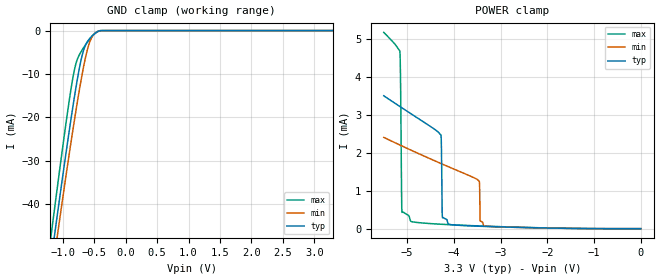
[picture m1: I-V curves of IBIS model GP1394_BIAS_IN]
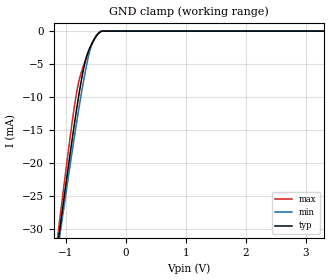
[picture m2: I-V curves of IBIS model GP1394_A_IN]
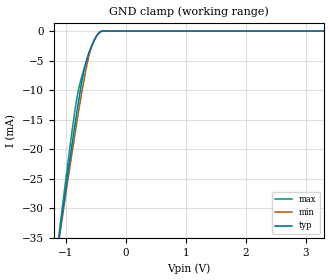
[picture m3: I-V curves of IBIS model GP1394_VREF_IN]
| TEXAS INSTRUMENTS INCORPORATED
| Standard Linear and Logic Group
| IBIS Model of SN74GTLP1394
| 2-Bit LVTTL-TO-GTLP Adjustable-Edge-Rate Bus Tran. with Split LVTTL Port
| This file contains package information for the following:
|  SOIC 16-pin (D) package as [Component] GTLP1394_D
|  TSSOP 16 pin (PW)  package as [Component] GTLP1394_PW
|  TVSOP 16 pin (DGV)  package as [Component] GTLP1394_DGV
| This device can be powered at the following Vccs:
|  3.3 volt Vcc
| This file provides unique models under the [Model Selector] for each Vcc.
| For operation at a specific Vcc, select the appropriate model after each
| [Model Selector] keyword.
[IBIS Ver]   3.2
[Comment char]  |_char
[File Name]   sn74gtlp1394.ibs
[File Rev]   1.1 | e_die
[Date]   January 31, 2001
[Source]   Data created from TI-SPICE simulations at TI-SLL.
[Notes]   The following is an IBIS list for the GTLP1394.
   Please contact sllibis@ti.com with questions and
   comments concerning SLL IBIS models.
   - We omitted PWR clamp curves from some input models,
   as there are no power clamp circuits there.
[Disclaimer] Property of Texas Instruments Incorporated.  Unauthorized
   reproduction and/or distribution is strictly prohibited.
   This product is protected under copyright law.
   Created  2001, (C) Copyright  2001, Texas Instruments
   Incorporated, All Rights Reserved
   UNLESS THERE IS A SIGNED, WRITTEN AGREEMENT TO THE
   CONTRARY, TEXAS INSTRUMENTS (TI) IS PROVIDING THE IBIS
   MODELS  AND WITHOUT ANY WARRANTY, EXPRESSED OR
   IMPLIED.  TI assumes no liability for:
   1) the accuracy of the IBIS models provided to your
   company;
   2) the proper functioning of these IBIS Models in your
   design or for any resulting applications; or
   3) infringement of patents, copyrights or intellectual
   property rights resulting from your use of these IBIS
   models.
   TI provides IBIS Models as a service to our customers.
   You and your company shall not distribute, sell or give
   these models to anyone else without prior written
   permission from TI.
   TI reserves the right to make changes to our products or
   to discontinue any semiconductor product or service
   without notice, and advises our customers to obtain the
   latest version of relevant information to verify, before
   placing orders, that the information being relied on is
   current.
   Please be aware that your receipt and use of the IBIS
   information provided shall serve as acceptance of these
   terms and conditions.  If you do not accept these terms,
   you should return or destroy the IBIS models and any
   other accompanying information immediately.
| Component GTLP1394_D 16-pin SOIC
[Component]   GTLP1394_D
[Manufacturer]   Texas Instruments, Inc.
[Package]
|   typ   min   max
R_pkg   3.900e-02   2.800e-02   4.900e-02
L_pkg   3.453e-09   2.350e-09   4.375e-09
C_pkg   5.210e-13   2.540e-13   7.080e-13
[Pin]   signal_name   model_name   R_pin   L_pin   C_pin
1   NOEBY   GP1394_NOEBY_IN   4.200e-02   4.336e-09   7.030e-13
2   Y1   GP1394_Y_OUT   4.900e-02   3.778e-09   6.340e-13
3   Y2   GP1394_Y_OUT   2.800e-02   3.449e-09   5.180e-13
4   VCC   POWER   2.900e-02   2.393e-09   2.540e-13
5   A1   GP1394_A_IN   2.800e-02   2.350e-09   2.640e-13
6   A2   GP1394_A_IN   4.800e-02   3.312e-09   4.830e-13
7   NOEAB   GP1394_NOEAB_IN   4.300e-02   3.629e-09   6.040e-13
8   NERC   GP1394_NERC_IN   4.400e-02   4.375e-09   7.080e-13
9   TNC   GP1394_TNC_IN   4.200e-02   4.336e-09   7.030e-13
10   VREF   GP1394_VREF_IN   4.900e-02   3.778e-09   6.340e-13
11   GND   GND   2.800e-02   3.449e-09   5.180e-13
12   B2   GP1394_B_IO   2.900e-02   2.393e-09   2.550e-13
13   GND   GND   2.800e-02   2.350e-09   2.640e-13
14   B1   GP1394_B_IO   4.800e-02   3.312e-09   4.830e-13
15   GND   GND   4.300e-02   3.629e-09   6.040e-13
16   BIASVCC   GP1394_BIAS_IN   4.400e-02   4.375e-09   7.080e-13
[Component]   GTLP1394_DGV
[Manufacturer]   Texas   Instruments,   Inc.
[Package]
|   typ   min   max
R_pkg   0.039   0.033   0.045
L_pkg   2.54E-09   2.32E-09   2.94E-09
C_pkg   3.86E-13   3.34E-13   4.49E-13
[Pin]   signal_name   model_name   R_pin   L_pin   C_pin
1   NOEBY   GP1394_NOEBY_IN   0.035   2.91E-09   4.17E-13
2   Y1   GP1394_Y_OUT   0.042   2.56E-09   4.46E-13
3   Y2   GP1394_Y_OUT   0.038   2.34E-09   3.45E-13
4   VCC   POWER   0.038   2.32E-09   3.34E-13
5   A1   GP1394_A_IN   0.039   2.32E-09   3.34E-13
6   A2   GP1394_A_IN   0.038   2.35E-09   3.42E-13
7   NOEAB   GP1394_NOEAB_IN   0.04   2.54E-09   4.41E-13
8   NERC   GP1394_NERC_IN   0.033   2.90E-09   4.18E-13
9   TNC   GP1394_TNC_IN   0.035   2.93E-09   4.19E-13
10   VREF   GP1394_VREF_IN   0.045   2.63E-09   4.49E-13
11   GND   GND   0.039   2.37E-09   3.47E-13
12   B2   GP1394_B_IO   0.039   2.33E-09   3.35E-13
13   GND   GND   0.039   2.32E-09   3.35E-13
14   B1   GP1394_B_IO   0.039   2.36E-09   3.45E-13
15   GND   GND   0.041   2.57E-09   4.46E-13
16   BIASVCC   GP1394_BIAS_IN   0.035   2.94E-09   4.20E-13
[Component]   GTLP1394_PW
[Manufacturer]   Texas   Instruments,   Inc.
[Package]
|   typ   min   max
R_pkg   0.045   0.038   0.051
L_pkg   2.59E-09   2.45E-09   3.08E-09
C_pkg   2.81E-13   2.43E-13   3.77E-13
[Pin]   signal_name   model_name   R_pin   L_pin   C_pin
1   NOEBY   GP1394_NOEBY_IN   0.04   3.08E-09   3.77E-13
2   Y1   GP1394_Y_OUT   0.038   2.46E-09   2.81E-13
3   Y2   GP1394_Y_OUT   0.051   2.51E-09   2.55E-13
4   VCC   POWER   0.051   2.45E-09   2.43E-13
5   A1   GP1394_A_IN   0.051   2.45E-09   2.43E-13
6   A2   GP1394_A_IN   0.051   2.51E-09   2.55E-13
7   NOEAB   GP1394_NOEAB_IN   0.038   2.46E-09   2.81E-13
8   NERC   GP1394_NERC_IN   0.04   3.08E-09   3.77E-13
9   TNC   GP1394_TNC_IN   0.039   2.83E-09   3.16E-13
10   VREF   GP1394_VREF_IN   0.038   2.46E-09   2.79E-13
11   GND   GND   0.051   2.51E-09   2.55E-13
12   B2   GP1394_B_IO   0.051   2.45E-09   2.43E-13
13   GND   GND   0.051   2.45E-09   2.43E-13
14   B1   GP1394_B_IO   0.051   2.51E-09   2.55E-13
15   GND   GND   0.038   2.46E-09   2.79E-13
16   BIASVCC   GP1394_BIAS_IN   0.039   2.83E-09   3.16E-13
| Models and submodels in the file (9): GP1394_BIAS_IN (Input), GP1394_A_IN (Input), GP1394_VREF_IN (Input), GP1394_TNC_IN (Input), GP1394_NOEAB_IN (Input), GP1394_NERC_IN (Input), GP1394_NOEBY_IN (Input), GP1394_B_IO (I/O_open_drain), GP1394_Y_OUT (3-state)
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| NOTE:  The [Diff Pin] section is commented out because the ibischk3 program
|   currently flags it as an Error when it shouldn't
| [Diff Pin]  inv_pin   vdiff   tdelay_typ
|14   10   100mv   NA
|12   10   100mv   NA
[Model]   GP1394_BIAS_IN
Model_type  Input
Vinl=0.8
Vinh=2.0
| variable   typ   min   max
C_comp   3.57pF   2.55pF   5.23pF
[Temperature Range]   40   100   -40
| Ambient temperature   25   85   -40
[Voltage range]   3.3   3.15   3.45
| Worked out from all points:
|   GND clamp passes 1 mA (typ) near -0.52 V on its own axis
|   POWER clamp passes 1 mA (typ) near -4.26 V on its own axis
[GND Clamp]
| GP1394_BIAS_IN
|   Voltage   I(typ)   I(min)   I(max)
-5.5V     -555.7mA   -541.3mA   -574.5mA
-1.225V   -57.07mA   -61.47mA   -51.46mA
-1.175V   -51.7mA    -56.27mA   -45.84mA
-1.125V   -46.38mA   -51.1mA    -40.26mA
-1.08V    -41.63mA   -46.5mA    -35.29mA
-895mV    -22.79mA   -28.11mA   -15.81mA
-800mV    -13.87mA   -19.21mA   -8.07mA
-720mV    -7.451mA   -12.24mA   -5.118mA
-655mV    -3.908mA   -7.249mA   -3.609mA
-570mV    -1.797mA   -2.547mA   -1.904mA
-475mV    -522.4uA   -477.6uA   -468.2uA
3.3V      252pA      960.1pA    1.676nA
[POWER Clamp]
| GP1394_BIAS_IN
|   Voltage   I(typ)   I(min)   I(max)
-5.5V     3.494mA    2.4mA      5.161mA
-5.155V   3.212mA    2.199mA    4.666mA
-5.14V    3.2mA      2.191mA    3.786mA
-5.11V    3.176mA    2.174mA    425.6uA
-4.92V    3.023mA    2.066mA    192.8uA
-4.275V   2.456mA    1.713mA    116.3uA
-4.245V   284.7uA    1.697mA    114.3uA
-4.115V   121.8uA    1.628mA    105.9uA
-3.455V   63.49uA    1.245mA    71.72uA
-3.44V    62.83uA    228.7uA    71.06uA
-3.345V   58.83uA    74.81uA    66.93uA
-95.1fV   252pA      945.3pA    1.705nA
[Model]   GP1394_A_IN
Model_type  Input
Vinl=0.8
Vinh=2.0
| variable   typ   min   max
C_comp   2.48pF   1.86pF   3.64pF
[Temperature Range]   40   100   -40
| Ambient temperature   25   85   -40
[Voltage range]   3.3   3.15   3.45
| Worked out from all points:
|   GND clamp passes 1 mA (typ) near -0.51 V on its own axis
[GND Clamp]
| GP1394_A_IN
|   Voltage   I(typ)   I(min)   I(max)
-5.5V     -355mA     -335.7mA   -380.8mA
-1.155V   -33.69mA   -34.48mA   -32.48mA
-1.115V   -30.96mA   -31.93mA   -29.51mA
-1.075V   -28.26mA   -29.39mA   -26.57mA
-895mV    -16.45mA   -18.27mA   -13.82mA
-840mV    -13.04mA   -15.02mA   -10.38mA
-795mV    -10.38mA   -12.44mA   -8.1mA
-690mV    -5.112mA   -6.847mA   -4.848mA
-605mV    -2.629mA   -3.201mA   -2.83mA
-535mV    -1.376mA   -1.322mA   -1.427mA
-445mV    -270.8uA   -216.6uA   -189uA
3.3V      184.4pA    833.1pA    1.235nA
[Model]   GP1394_VREF_IN
Model_type  Input
Vinl=0.8
Vinh=2.0
| variable   typ   min   max
C_comp   4.23pF   3.29pF   4.82pF
[Temperature Range]   40   100   -40
| Ambient temperature   25   85   -40
[Voltage range]   3.3   3.15   3.45
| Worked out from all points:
|   GND clamp passes 1 mA (typ) near -0.49 V on its own axis
[GND Clamp]
| GP1394_VREF_IN
|   Voltage   I(typ)   I(min)   I(max)
-5.5V     -396.3mA   -371.4mA   -429.5mA
-1.12V    -35.63mA   -35.94mA   -34.96mA
-1.08V    -32.62mA   -33.14mA   -31.64mA
-890mV    -18.76mA   -20.22mA   -16.49mA
-835mV    -14.97mA   -16.65mA   -12.62mA
-790mV    -12.01mA   -13.81mA   -10.03mA
-735mV    -8.682mA   -10.48mA   -7.756mA
-685mV    -6.129mA   -7.664mA   -6.055mA
-600mV    -3.233mA   -3.656mA   -3.472mA
-530mV    -1.653mA   -1.549mA   -1.684mA
-435mV    -224.9uA   -193.5uA   -124.6uA
3.3V      334pA      1.329nA    1.856nA
